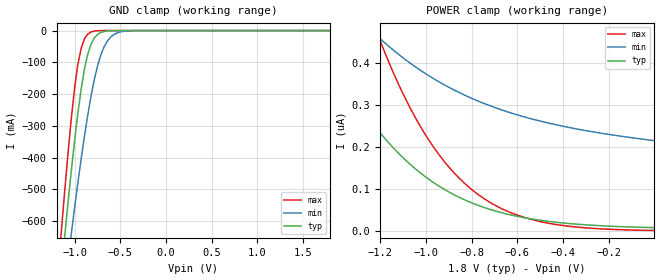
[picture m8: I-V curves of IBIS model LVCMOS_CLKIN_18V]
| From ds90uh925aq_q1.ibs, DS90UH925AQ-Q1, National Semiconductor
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[Model] LVCMOS_CLKIN_18V
Model_type Input
Vinh = 1.17V
Vinl = 0.62V
C_comp   6.98pF   6.05pF   8.06pF
[Voltage Range]   1.8V   1.62V   1.98V
[Temperature Range]   25.0   130.0   -40.0
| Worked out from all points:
|   GND clamp passes 1 mA (typ) near -0.64 V on its own axis
[GND Clamp]
-1.8V     -2.96A     -2.635A    -3.228A
-1.147V   -756.8mA   -899mA     -630.1mA
-1.114V   -658.8mA   -819.7mA   -517.7mA
-1.076V   -548.3mA   -728.9mA   -393.4mA
-1.039V   -442.8mA   -640.4mA   -278.7mA
-968.4mV  -265.6mA   -483.8mA   -110.5mA
-892.8mV  -119mA     -330.2mA   -25.29mA
-822.6mV  -43.25mA   -207.4mA   -4.329mA
-747mV    -11.35mA   -107.3mA   -370.4uA
-676.8mV  -2.58mA    -49.95mA   -28.17uA
-493.2mV  -19.23uA   -3.72mA    -1.533uA
1.796V    8.086nA    0A         608.3pA
[POWER Clamp]
-1.8V     914.6nA    909.1nA    12.77uA
-1.487V   484.9nA    632.4nA    976.4nA
-1.341V   340.7nA    534.4nA    679.3nA
-1.255V   271.3nA    485.1nA    533.2nA
-1.217V   244.4nA    465.5nA    476.2nA
-1.109V   179nA      415.6nA    336.1nA
-1.001V   128.6nA    374.1nA    227.9nA
-887.4mV  89.46nA    338.5nA    144.8nA
-763.2mV  59.54nA    307.4nA    83.79nA
-633.6mV  39.05nA    282nA      45.02nA
-487.8mV  24.86nA    260.1nA    21.31nA
-1.8mV    8.155nA    215.3nA    1.483nA
